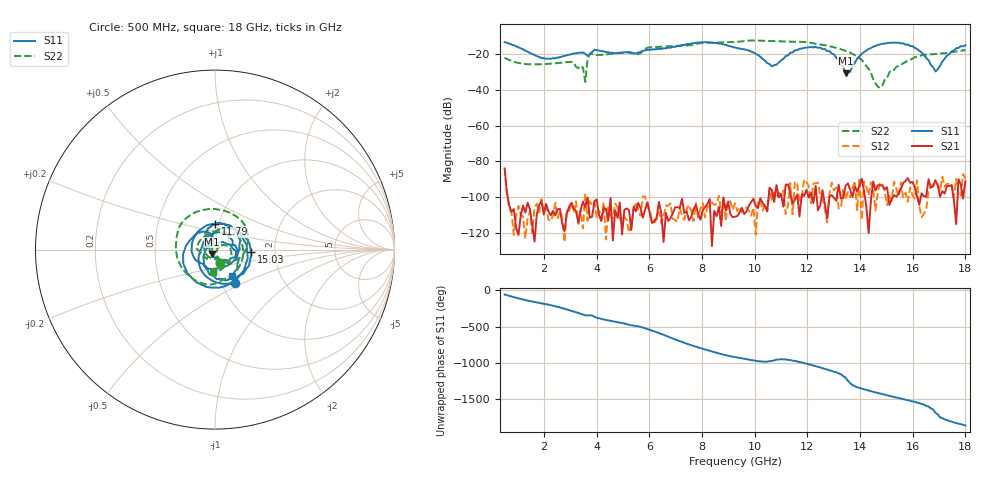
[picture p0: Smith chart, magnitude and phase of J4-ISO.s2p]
!Agilent Technologies,N5230C,MY49001096,A.09.42.15
!Agilent N5230C: A.09.42.15
!Date: Thursday, June 29, 2023 09:46:48
!Correction: S11(Full 2 Port(1,2))
!S21(Full 2 Port(1,2))
!S12(Full 2 Port(1,2))
!S22(Full 2 Port(1,2))
!S2P File: Measurements: S11, S21, S12, S22:
# Hz S  dB  R 50
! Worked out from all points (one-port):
!   201 points, 500 MHz to 18 GHz, reference 50 ohm
!   lowest |S11| = -30.7 dB at 13.45 GHz (marker M1), VSWR 1.06, Z = 48.4 - j2.4 ohm
!   |S11| at or under -10 dB: start of sweep to end of sweep
!   S11 on the Smith chart (normalised r, x): 500 MHz: 1.15, -0.44; 11.79 GHz: 0.97, +0.28; 15.03 GHz: 1.50, -0.04; 18 GHz: 1.16, -0.35
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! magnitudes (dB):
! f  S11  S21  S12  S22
! 500 MHz  -13.4  -83.8  -83.9  -22.1
! 2.075 GHz  -22.7  -103.7  -104.6  -25.6
! 3.475 GHz  -19.1  -102.4  -117.3  -27.6
! 3.562 GHz  -19.9  -105.5  -97.8  -35.6
! 3.65 GHz  -21.1  -100.2  -113.1  -23.2
! 3.737 GHz  -20.1  -111.4  -102.2  -19.8
! 6.362 GHz  -17.2  -102.6  -108.2  -16.0
! 8.025 GHz  -13.4  -107.3  -103.2  -14.0
! 9.25 GHz  -16.4  -110.8  -103.4  -13.2
! 10.65 GHz  -26.9  -95.9  -101.4  -12.8
! 11.79 GHz  -17.0  -98.2  -99.9  -13.3
! 12.22 GHz  -16.3  -103.2  -92.4  -14.0
! 13.01 GHz  -20.2  -100.3  -96.2  -16.3
! 13.45 GHz  -30.7  -93.5  -101.0  -18.3
! 14.06 GHz  -19.9  -89.7  -112.5  -23.3
! 14.68 GHz  -14.9  -93.3  -97.2  -38.3
! 15.03 GHz  -13.9  -94.3  -104.4  -33.4
! 15.11 GHz  -13.8  -104.3  -99.3  -30.3
! 16.16 GHz  -17.1  -99.5  -90.6  -21.5
! 16.86 GHz  -29.8  -90.5  -93.1  -20.0
! 17.48 GHz  -18.6  -93.3  -92.3  -19.0
! 18 GHz  -15.1  -91.0  -89.8  -18.0
